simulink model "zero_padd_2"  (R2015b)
settings: Solver=ode45  StartTime=0.0  StopTime=100  RelTol=1e-3
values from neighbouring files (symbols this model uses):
  fs = 4000    [abtast_rate_1.m]    (also in ad_test_12.m = ',     num2str(fs),'; ad_test_2.m = ',     num2str(fs),'; ad_test_3.m = ',     num2str(fs),'; DA_wandler_spektr_1.m = 100)
  fsig1 = 100.5    [leakage_3.m]    (also in leakage_4.m; zero_padd1.m = 100; zero_padd2.m = 100; zero_padd3.m = 100)
  fsig2 = 150.3    [leakage_3.m]    (also in leakage_4.m; zero_padd1.m = ',num2str(fsig2),' Hz und N = ',     num2str(N),' bzw. nfft ; zero_padd2.m = ',num2str(fsig2),' Hz und N = ',     num2str(N),' bzw. nfft ; zero_padd3.m = ',num2str(fsig2),' Hz und N = ',     num2str(N),' bzw. nfft )
  N = 4*1024    (= 4096)    [ad_test_12.m]    (also in ad_test_2.m; ad_test_3.m; DA_wandler_spektr_1.m = 1000; DA_wandler_spektr_2.m = 1024)
  nfft = 2^p2    [DA_wandler_spektr_1.m]    (also in DA_wandler_spektr_2.m; PSD_korrelation_1.m = 2^(nextpow2(2*lag_max)); welch_1.m = 256; zero_padd1.m = ',num2str(nfft),')
  pw = sum(hanning(N).^2)/N    [leakage_2.m]    (also in leakage_3.m; leakage_4.m; welch_1.m = sum(hamming(nfft).^2)/nfft; zero_padd2.m = sum(hamming(N).^2)/N)
undefined symbols (not defined in the file or in its folder): Fs, get
libraries: dspspect3 x1, dspstat3 x1, dspsnks4 x1, dspsigops x1

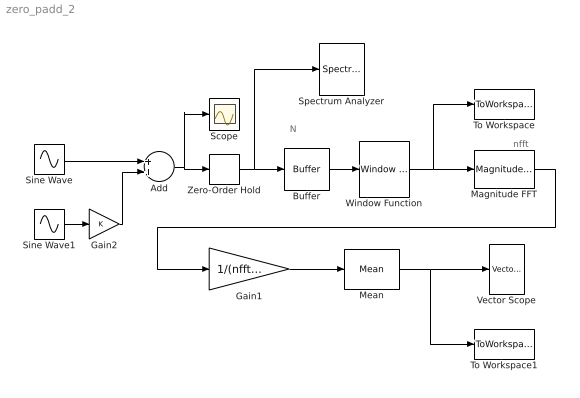
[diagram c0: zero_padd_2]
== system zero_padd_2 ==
  note: nfft
  note: N
  Add : Sum
  Buffer : Buffer  N=N  TreatMby1Signals=One channel
  Gain1 : Gain  Gain=1/(nfft*N*pw)
  Gain2 : Gain
  Magnitude FFT : dspspect3/Magnitude FFT  mag_or_magsq=Magnitude squared  FFTImplementation=Auto  fftLenInherit=off  fftsize=nfft  WrapInput=on
  Mean : dspstat3/Mean  run=on  reset_popup=None  directionMode=Each column  dimension=1  roiEnable=off  roiType=Rectangles  roiPortion=Entire ROI  roiOutput=Individual statistics for each ROI  roiFlag=off  outputDataTypeStr=Inherit: Same as accumulator  outputLastDataTypeStr=Inherit: Same as accumulator  outputMin=[]  outputMax=[]  roundingMode=Floor  overflowMode=off
  Scope : Scope
  Sine Wave : Sin  Frequency=2*pi*fsig1  SampleTime=0
  Sine Wave1 : Sin  Frequency=2*pi*fsig2  SampleTime=0
  Spectrum Analyzer : SpectrumAnalyzer
  To Workspace : ToWorkspace  VariableName=y  SaveFormat=Structure  SampleTime=-1
  To Workspace1 : ToWorkspace  VariableName=Y  SaveFormat=Structure  SampleTime=-1
  Vector Scope : dspsnks4/Vector Scope  ScopeProperties=on  Domain=Frequency  HorizSpan=1  DisplayProperties=off  AxisGrid=on  Memory=off  FrameNumber=on  AxisLegend=off  AxisZoom=off  OpenScopeAtSimStart=on  OpenScopeImmediately=off  FigPos=get(0,'defaultfigureposition')  AxisProperties=off  XUnits=Hertz  XRange=[-Fs/2...Fs/2]  InheritXIncr=off  XIncr=1/1000  XLabel=Time  XLimit=User-defined  XMin=-500  XMax=500  XStart=0  YUnits=dB  YLabel=Amplitude  LineProperties=off  XAxisParamsVer=6.9
  Window Function : dspsigops/Window Function  winmode=Apply window to input  wintype=Hamming  sampmode=Continuous  samptime=1  N=64  Rs=50  beta=10  winsamp=Symmetric  UserWindow=hamming  OptParams=off  UserParams={'symmetric'}  dataType=double  isSigned=on  wordLen=16  udDataType=sfix(16)  fracBitsMode=Best precision  numFracBits=15  roundingMode=Floor  overflowMode=off  numSidelobes=4  sidelobeLevel=-30
  Zero-Order Hold : ZeroOrderHold  SampleTime=1/fs
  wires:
  Zero-Order Hold/1 -> Spectrum Analyzer/1, Buffer/1
  Buffer/1 -> Window Function/1
  Magnitude FFT/1 -> Gain1/1
  Window Function/1 -> Magnitude FFT/1, To Workspace/1
  Gain1/1 -> Mean/1
  Add/1 -> Scope/1, Zero-Order Hold/1
  Sine Wave/1 -> Add/1
  Sine Wave1/1 -> Gain2/1
  Gain2/1 -> Add/2
  Mean/1 -> Vector Scope/1, To Workspace1/1
